FUNCTION "SFOGLIATORE" : VOID
TITLE =COMANDO SFOGLIATORE
AUTHOR : LD
FAMILY : DESTACK
NAME : SFOGL
VERSION : 0.1

BEGIN
NETWORK
TITLE =Sicurezze per sfogliatore
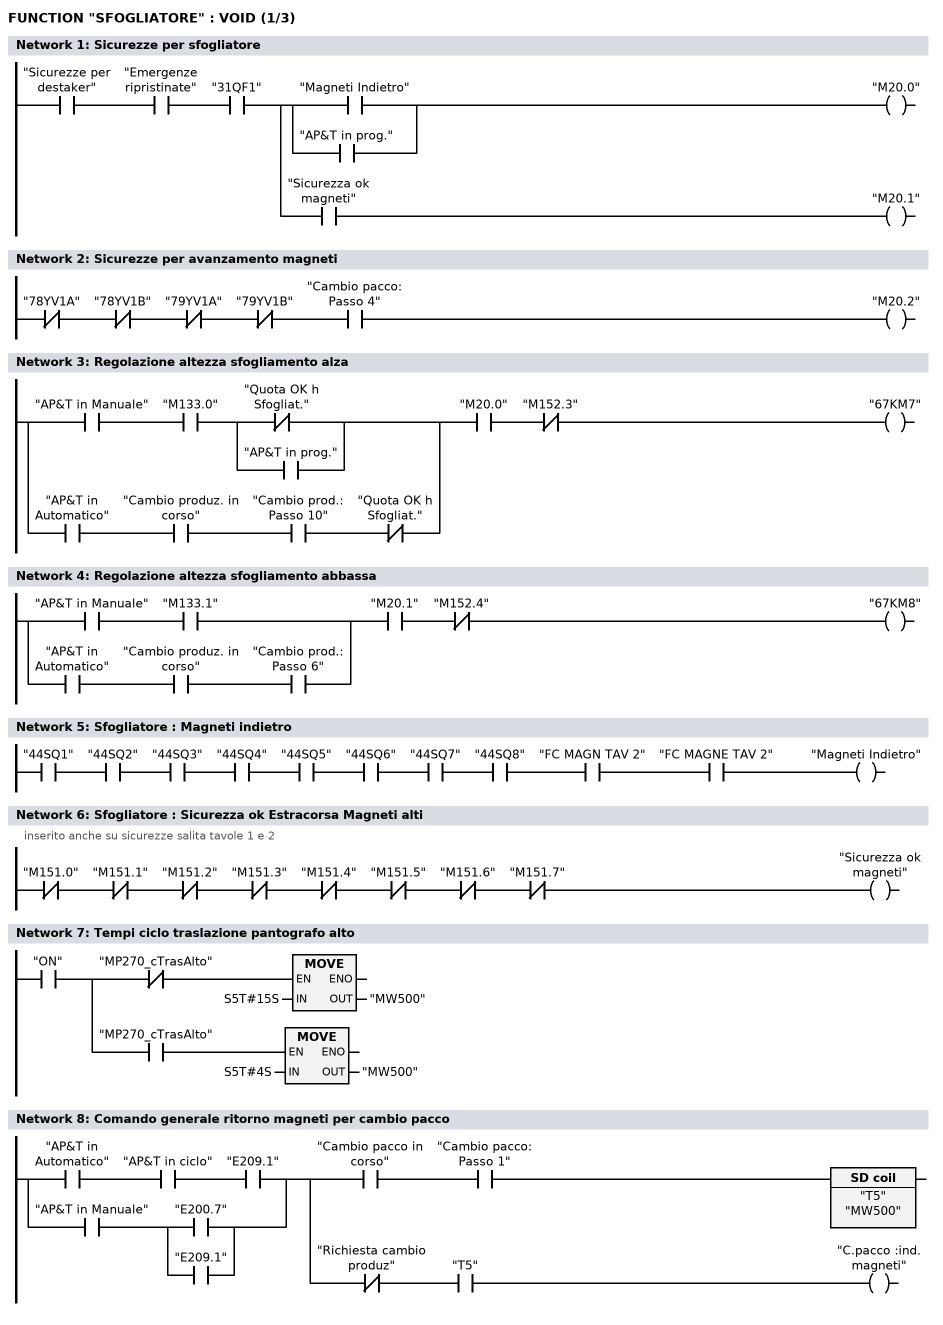
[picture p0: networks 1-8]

      U     "Sicurezze per destaker";
      U     "Emergenze ripristinate";
      U     "31QF1";
      =     L      0.0;
      U     L      0.0;
      U(    ;
      O     "Magneti Indietro";
      O     "AP&T in prog.";
      )     ;
      =     "M20.0";
      U     L      0.0;
      U     "Sicurezza ok magneti";
      =     "M20.1";
NETWORK
TITLE =Sicurezze per avanzamento magneti

      UN    "78YV1A";
      UN    "78YV1B";
      UN    "79YV1A";
      UN    "79YV1B";
      U     "Cambio pacco: Passo 4";
      =     "M20.2";
NETWORK
TITLE =Regolazione altezza sfogliamento alza

      U(    ;
      U     "AP&T in Manuale";
      U     "M133.0";
      U(    ;
      ON    "Quota OK h Sfogliat.";
      O     "AP&T in prog.";
      )     ;
      O     ;
      U     "AP&T in Automatico";
      U     "Cambio produz. in corso";
      U     "Cambio prod.: Passo 10";
      UN    "Quota OK h Sfogliat.";
      )     ;
      U     "M20.0";
      UN    "M152.3";
      =     "67KM7";
NETWORK
TITLE =Regolazione altezza sfogliamento abbassa

      U(    ;
      U     "AP&T in Manuale";
      U     "M133.1";
      O     ;
      U     "AP&T in Automatico";
      U     "Cambio produz. in corso";
      U     "Cambio prod.: Passo 6";
      )     ;
      U     "M20.1";
      UN    "M152.4";
      =     "67KM8";
NETWORK
TITLE =Sfogliatore : Magneti indietro

      U     "44SQ1";
      U     "44SQ2";
      U     "44SQ3";
      U     "44SQ4";
      U     "44SQ5";
      U     "44SQ6";
      U     "44SQ7";
      U     "44SQ8";
      U     "FC MAGN TAV 2";
      U     "FC MAGNE TAV 2";
      =     "Magneti Indietro";
NETWORK
TITLE =Sfogliatore : Sicurezza ok Estracorsa Magneti alti
//inserito anche su sicurezze salita tavole 1 e 2
      UN    "M151.0";
      UN    "M151.1";
      UN    "M151.2";
      UN    "M151.3";
      UN    "M151.4";
      UN    "M151.5";
      UN    "M151.6";
      UN    "M151.7";
      =     "Sicurezza ok magneti";
NETWORK
TITLE =Tempi ciclo traslazione pantografo alto

      U     "ON";
      =     L      0.0;
      U     L      0.0;
      UN    "MP270_cTrasAlto";
      SPBNB _001;
      L     S5T#15S;
      T     "MW500";
_001: NOP   0;
      U     L      0.0;
      U     "MP270_cTrasAlto";
      SPBNB _002;
      L     S5T#4S;
      T     "MW500";
_002: NOP   0;
NETWORK
TITLE =Comando generale ritorno magneti per cambio pacco

      U     "AP&T in Automatico";
      U     "AP&T in ciclo";
      U     "E209.1";
      O     ;
      U     "AP&T in Manuale";
      U(    ;
      O     "E200.7";
      O     "E209.1";
      )     ;
      =     L      0.0;
      U     L      0.0;
      U     "Cambio pacco in corso";
      U     "Cambio pacco: Passo 1";
      L     "MW500";
      SE    "T5";
      U     L      0.0;
      UN    "Richiesta cambio produz";
      U     "T5";
      =     "C.pacco :ind. magneti";
NETWORK
TITLE =Sfogliatore : Comando Impulso vuoto per ripristino prelievo
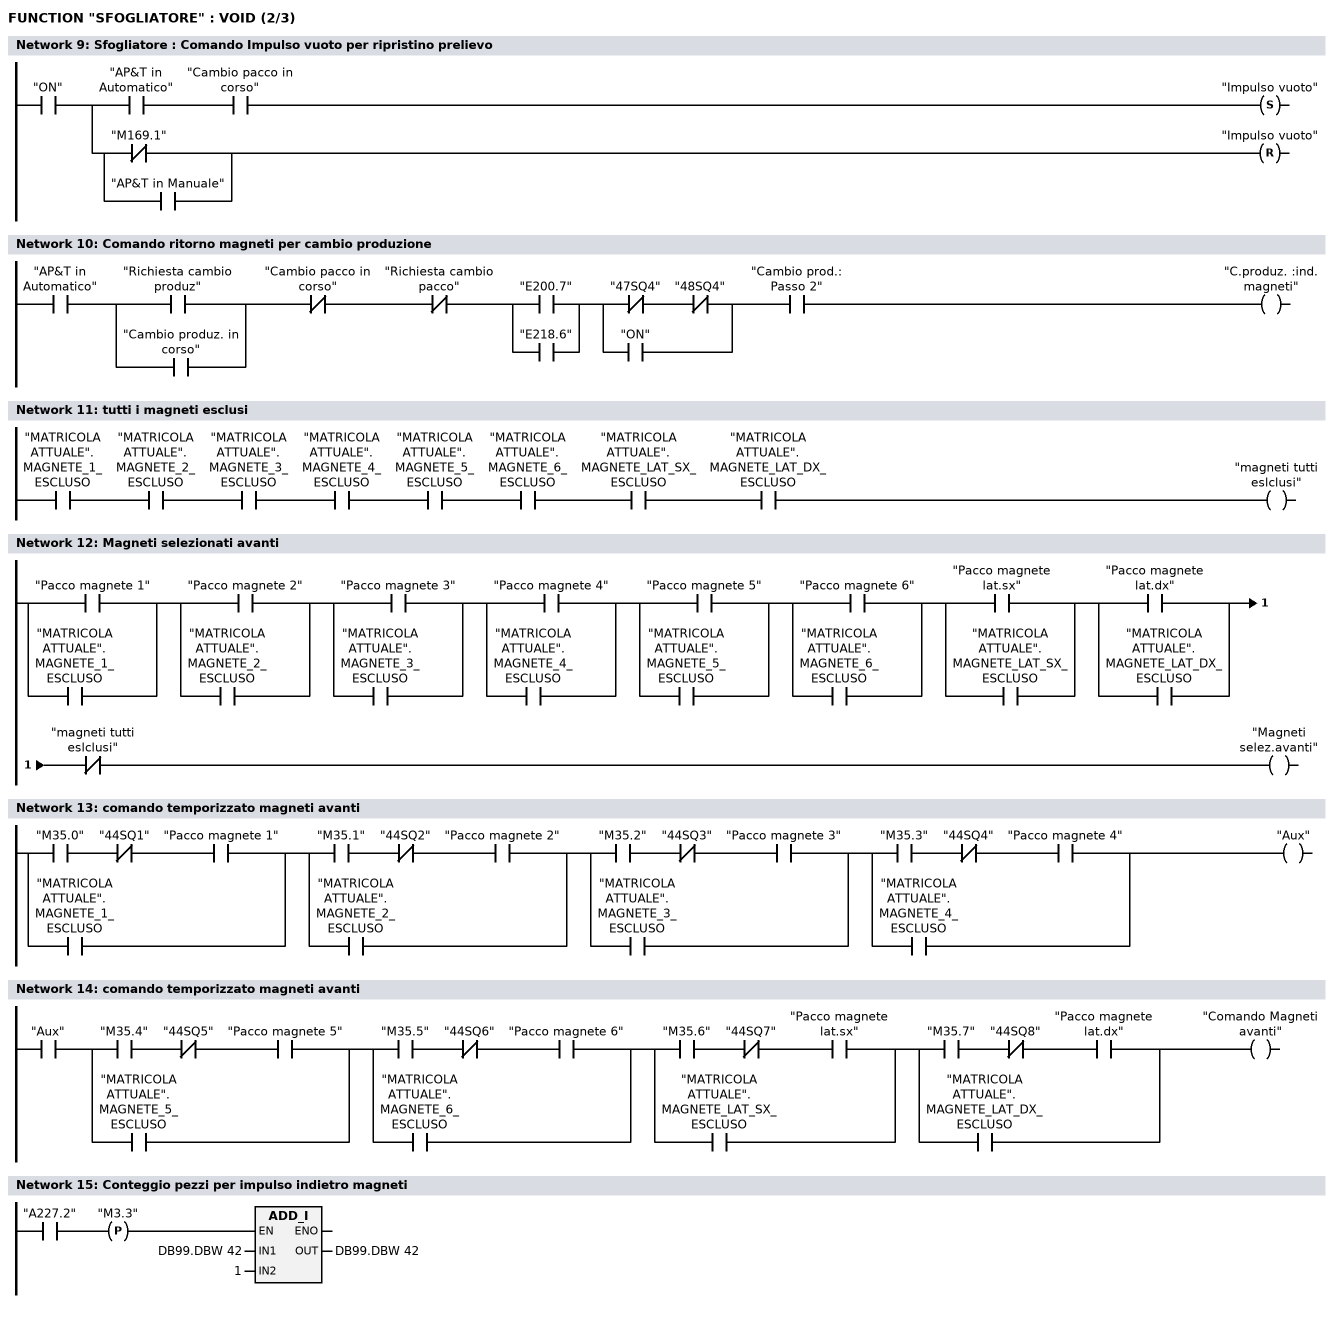
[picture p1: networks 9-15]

      U     "ON";
      =     L      0.0;
      U     L      0.0;
      U     "AP&T in Automatico";
      U     "Cambio pacco in corso";
      S     "Impulso vuoto";
      U     L      0.0;
      U(    ;
      ON    "M169.1";
      O     "AP&T in Manuale";
      )     ;
      R     "Impulso vuoto";
NETWORK
TITLE =Comando ritorno magneti per cambio produzione

      U     "AP&T in Automatico";
      U(    ;
      O     "Richiesta cambio produz";
      O     "Cambio produz. in corso";
      )     ;
      UN    "Cambio pacco in corso";
      UN    "Richiesta cambio pacco";
      U(    ;
      O     "E200.7";
      O     "E218.6";
      )     ;
      U(    ;
      UN    "47SQ4";
      UN    "48SQ4";
      O     "ON";
      )     ;
      U     "Cambio prod.: Passo 2";
      =     "C.produz. :ind. magneti";
NETWORK
TITLE =tutti i magneti esclusi



      U     "MATRICOLA ATTUALE".MAGNETE_1_ESCLUSO;
      U     "MATRICOLA ATTUALE".MAGNETE_2_ESCLUSO;
      U     "MATRICOLA ATTUALE".MAGNETE_3_ESCLUSO;
      U     "MATRICOLA ATTUALE".MAGNETE_4_ESCLUSO;
      U     "MATRICOLA ATTUALE".MAGNETE_5_ESCLUSO;
      U     "MATRICOLA ATTUALE".MAGNETE_6_ESCLUSO;
      U     "MATRICOLA ATTUALE".MAGNETE_LAT_SX_ESCLUSO;
      U     "MATRICOLA ATTUALE".MAGNETE_LAT_DX_ESCLUSO;
      =     "magneti tutti eslclusi";
NETWORK
TITLE =Magneti selezionati avanti

      U(    ;
      O     "Pacco magnete 1";
      O     "MATRICOLA ATTUALE".MAGNETE_1_ESCLUSO;
      )     ;
      U(    ;
      O     "Pacco magnete 2";
      O     "MATRICOLA ATTUALE".MAGNETE_2_ESCLUSO;
      )     ;
      U(    ;
      O     "Pacco magnete 3";
      O     "MATRICOLA ATTUALE".MAGNETE_3_ESCLUSO;
      )     ;
      U(    ;
      O     "Pacco magnete 4";
      O     "MATRICOLA ATTUALE".MAGNETE_4_ESCLUSO;
      )     ;
      U(    ;
      O     "Pacco magnete 5";
      O     "MATRICOLA ATTUALE".MAGNETE_5_ESCLUSO;
      )     ;
      U(    ;
      O     "Pacco magnete 6";
      O     "MATRICOLA ATTUALE".MAGNETE_6_ESCLUSO;
      )     ;
      U(    ;
      O     "Pacco magnete lat.sx";
      O     "MATRICOLA ATTUALE".MAGNETE_LAT_SX_ESCLUSO;
      )     ;
      U(    ;
      O     "Pacco magnete lat.dx";
      O     "MATRICOLA ATTUALE".MAGNETE_LAT_DX_ESCLUSO;
      )     ;
      UN    "magneti tutti eslclusi";
      =     "Magneti selez.avanti";
NETWORK
TITLE =comando temporizzato magneti avanti

      U(    ;
      U     "M35.0";
      UN    "44SQ1";
      U     "Pacco magnete 1";
      O     "MATRICOLA ATTUALE".MAGNETE_1_ESCLUSO;
      )     ;
      U(    ;
      U     "M35.1";
      UN    "44SQ2";
      U     "Pacco magnete 2";
      O     "MATRICOLA ATTUALE".MAGNETE_2_ESCLUSO;
      )     ;
      U(    ;
      U     "M35.2";
      UN    "44SQ3";
      U     "Pacco magnete 3";
      O     "MATRICOLA ATTUALE".MAGNETE_3_ESCLUSO;
      )     ;
      U(    ;
      U     "M35.3";
      UN    "44SQ4";
      U     "Pacco magnete 4";
      O     "MATRICOLA ATTUALE".MAGNETE_4_ESCLUSO;
      )     ;
      =     "Aux";
NETWORK
TITLE =comando temporizzato magneti avanti

      U     "Aux";
      U(    ;
      U     "M35.4";
      UN    "44SQ5";
      U     "Pacco magnete 5";
      O     "MATRICOLA ATTUALE".MAGNETE_5_ESCLUSO;
      )     ;
      U(    ;
      U     "M35.5";
      UN    "44SQ6";
      U     "Pacco magnete 6";
      O     "MATRICOLA ATTUALE".MAGNETE_6_ESCLUSO;
      )     ;
      U(    ;
      U     "M35.6";
      UN    "44SQ7";
      U     "Pacco magnete lat.sx";
      O     "MATRICOLA ATTUALE".MAGNETE_LAT_SX_ESCLUSO;
      )     ;
      U(    ;
      U     "M35.7";
      UN    "44SQ8";
      U     "Pacco magnete lat.dx";
      O     "MATRICOLA ATTUALE".MAGNETE_LAT_DX_ESCLUSO;
      )     ;
      =     "Comando Magneti avanti";
NETWORK
TITLE =Conteggio pezzi per impulso indietro magneti

      U     "A227.2";
      FP    "M3.3";
      SPBNB _003;
      L     DB99.DBW   42;
      L     1;
      +I    ;
      T     DB99.DBW   42;
_003: NOP   0;
NETWORK
TITLE =Aux impulso per magneti indietro
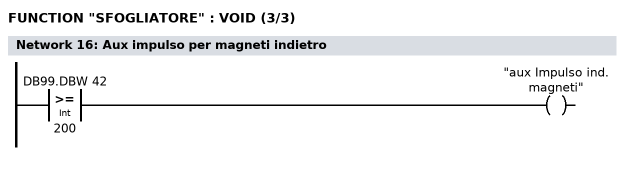
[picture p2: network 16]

      L     DB99.DBW   42;
      L     200;
      >=I   ;
      =     "aux Impulso ind. magneti";
NETWORK
TITLE =Memoria magneti avanti

      U(    ;
      O     "Comando Magneti avanti";
      O(    ;
      U     "Cambio pacco in corso";
      U     "Cambio pacco: Passo 4";
      UN    "Magneti Indietro";
      L     S5T#10S;
      SE    "T12";
      NOP   0;
      NOP   0;
      NOP   0;
      U     "T12";
      )     ;
      O     ;
      U(    ;
      O     "AP&T in Manuale";
      O     "Singolo";
      )     ;
      UN    "Cambio pacco in corso";
      UN    "Magneti Indietro";
      )     ;
      S     "M39.5";
      U     "Magneti Indietro";
      R     "M39.5";
      U     "M39.5";
      L     S5T#100MS;
      SE    "T6";
NETWORK
TITLE =
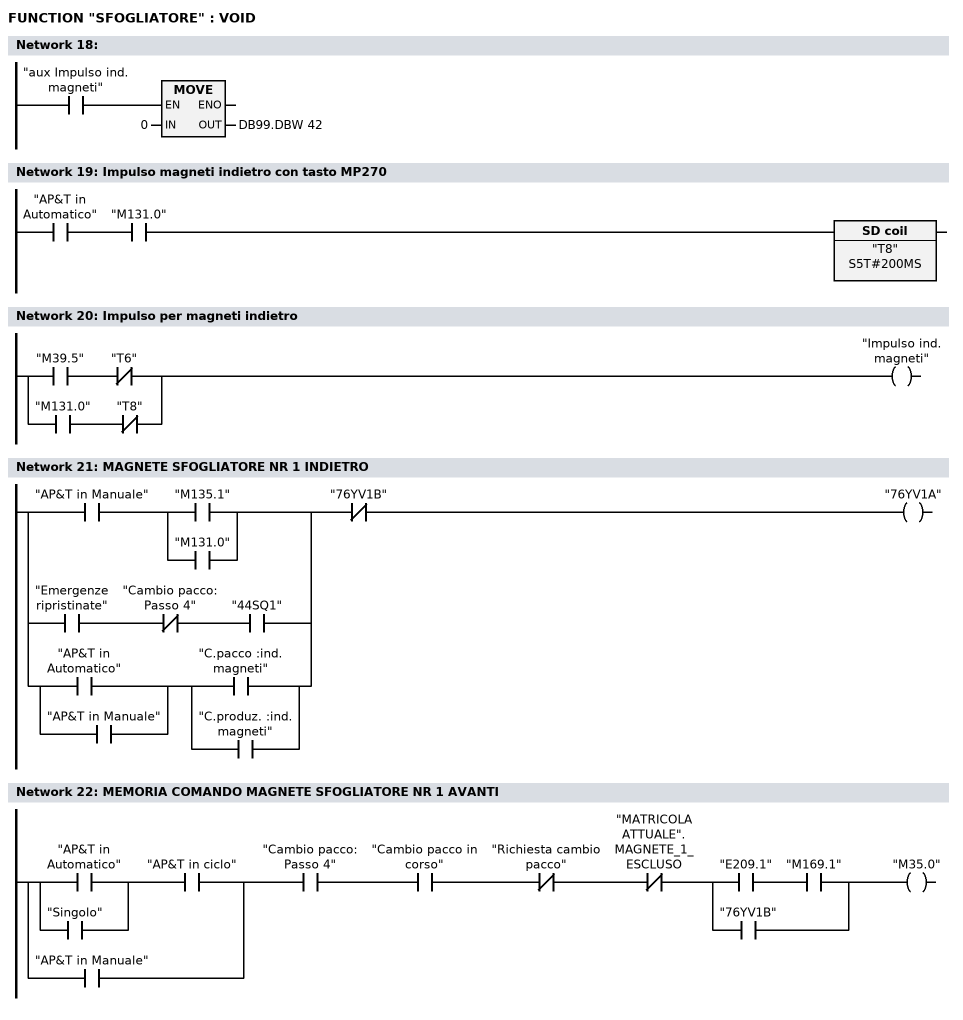
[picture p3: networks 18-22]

      U     "aux Impulso ind. magneti";
      SPBNB _004;
      L     0;
      T     DB99.DBW   42;
_004: NOP   0;
NETWORK
TITLE =Impulso magneti indietro con tasto MP270

      U     "AP&T in Automatico";
      U     "M131.0";
      L     S5T#200MS;
      SE    "T8";
NETWORK
TITLE =Impulso per magneti indietro

      U     "M39.5";
      UN    "T6";
      O     ;
      U     "M131.0";
      UN    "T8";
      =     "Impulso ind. magneti";
NETWORK
TITLE =MAGNETE SFOGLIATORE NR 1 INDIETRO

      U(    ;
      U     "AP&T in Manuale";
      U(    ;
      O     "M135.1";
      O     "M131.0";
      )     ;
      O     ;
      U     "Emergenze ripristinate";
      UN    "Cambio pacco: Passo 4";
      U     "44SQ1";
      O     ;
      U(    ;
      O     "AP&T in Automatico";
      O     "AP&T in Manuale";
      )     ;
      U(    ;
      O     "C.pacco :ind. magneti";
      O     "C.produz. :ind. magneti";
      )     ;
      )     ;
      UN    "76YV1B";
      =     "76YV1A";
NETWORK
TITLE =MEMORIA COMANDO MAGNETE SFOGLIATORE NR 1 AVANTI

      U(    ;
      U(    ;
      O     "AP&T in Automatico";
      O     "Singolo";
      )     ;
      U     "AP&T in ciclo";
      O     "AP&T in Manuale";
      )     ;
      U     "Cambio pacco: Passo 4";
      U     "Cambio pacco in corso";
      UN    "Richiesta cambio pacco";
      UN    "MATRICOLA ATTUALE".MAGNETE_1_ESCLUSO;
      U(    ;
      U     "E209.1";
      U     "M169.1";
      O     "76YV1B";
      )     ;
      =     "M35.0";
NETWORK
TITLE =COMANDO MAGNETE SFOGLIATORE NR 1 AVANTI

      O(    ;
      U(    ;
      U(    ;
      O     "AP&T in Automatico";
      O     "Singolo";
      )     ;
      U     "AP&T in ciclo";
      O     "AP&T in Manuale";
      )     ;
      U     "M35.0";
      U     "M20.2";
      UN    "Pacco magnete 1";
      L     S5T#500MS;
      SA    "M1_RitAvanti";
      NOP   0;
      NOP   0;
      NOP   0;
      U     "M1_RitAvanti";
      )     ;
      O     ;
      U(    ;
      O     "AP&T in Manuale";
      O     "AP&T in prog.";
      )     ;
      U(    ;
      O     "M135.0";
      O     ;
      U     "M137.4";
      UN    "MATRICOLA ATTUALE".MAGNETE_1_ESCLUSO;
      )     ;
      =     "76YV1B";
NETWORK
TITLE =MAGNETE SFOGLIATORE NR 2 INDIETRO
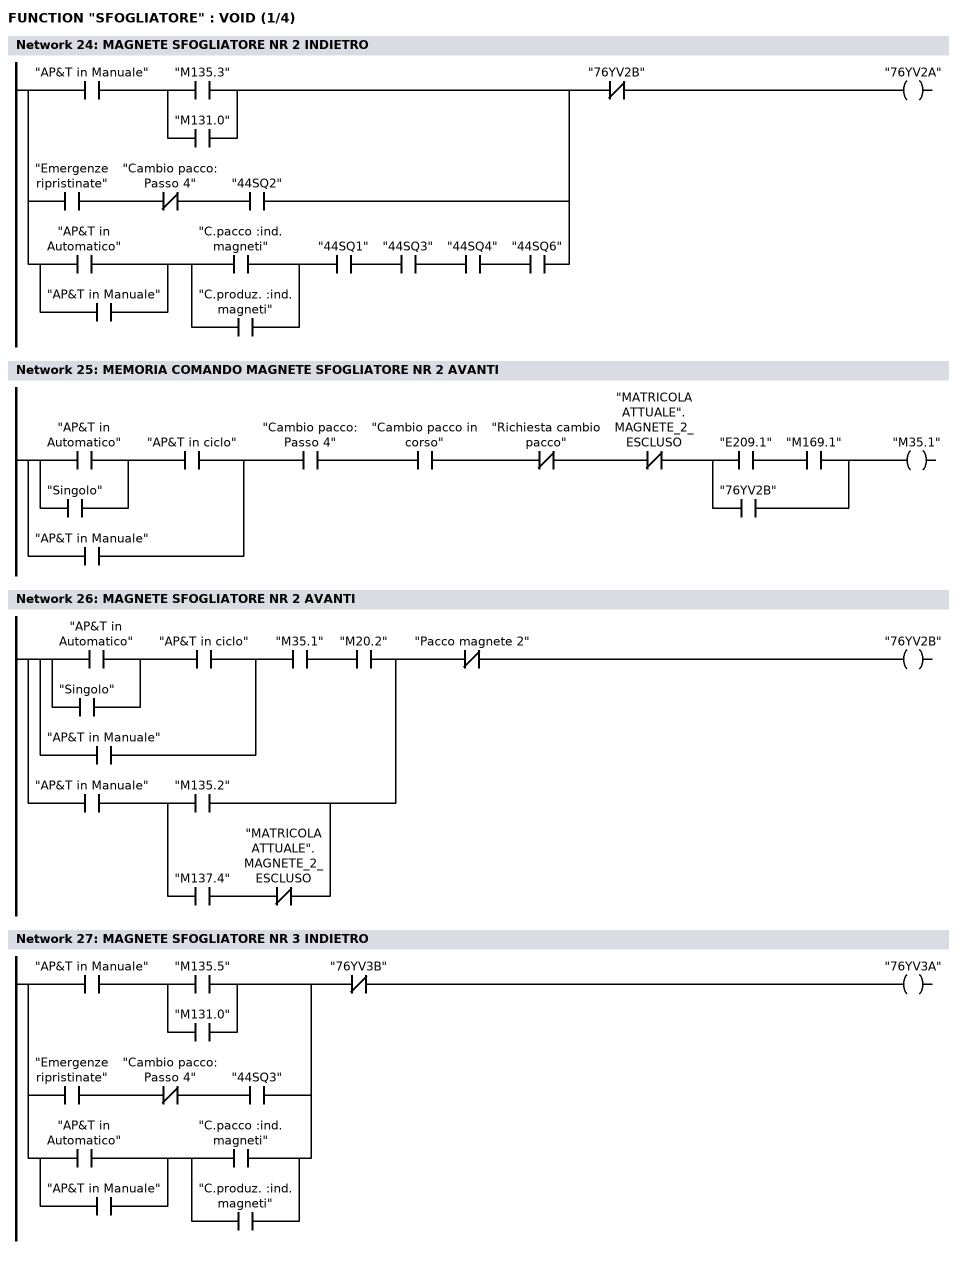
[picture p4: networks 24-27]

      U(    ;
      U     "AP&T in Manuale";
      U(    ;
      O     "M135.3";
      O     "M131.0";
      )     ;
      O     ;
      U     "Emergenze ripristinate";
      UN    "Cambio pacco: Passo 4";
      U     "44SQ2";
      O     ;
      U(    ;
      O     "AP&T in Automatico";
      O     "AP&T in Manuale";
      )     ;
      U(    ;
      O     "C.pacco :ind. magneti";
      O     "C.produz. :ind. magneti";
      )     ;
      U     "44SQ1";
      U     "44SQ3";
      U     "44SQ4";
      U     "44SQ6";
      )     ;
      UN    "76YV2B";
      =     "76YV2A";
NETWORK
TITLE =MEMORIA COMANDO MAGNETE SFOGLIATORE NR 2 AVANTI

      U(    ;
      U(    ;
      O     "AP&T in Automatico";
      O     "Singolo";
      )     ;
      U     "AP&T in ciclo";
      O     "AP&T in Manuale";
      )     ;
      U     "Cambio pacco: Passo 4";
      U     "Cambio pacco in corso";
      UN    "Richiesta cambio pacco";
      UN    "MATRICOLA ATTUALE".MAGNETE_2_ESCLUSO;
      U(    ;
      U     "E209.1";
      U     "M169.1";
      O     "76YV2B";
      )     ;
      =     "M35.1";
NETWORK
TITLE =MAGNETE SFOGLIATORE NR 2 AVANTI

      U(    ;
      U(    ;
      U(    ;
      O     "AP&T in Automatico";
      O     "Singolo";
      )     ;
      U     "AP&T in ciclo";
      O     "AP&T in Manuale";
      )     ;
      U     "M35.1";
      U     "M20.2";
      O     ;
      U     "AP&T in Manuale";
      U(    ;
      O     "M135.2";
      O     ;
      U     "M137.4";
      UN    "MATRICOLA ATTUALE".MAGNETE_2_ESCLUSO;
      )     ;
      )     ;
      UN    "Pacco magnete 2";
      =     "76YV2B";
NETWORK
TITLE =MAGNETE SFOGLIATORE NR 3 INDIETRO

      U(    ;
      U     "AP&T in Manuale";
      U(    ;
      O     "M135.5";
      O     "M131.0";
      )     ;
      O     ;
      U     "Emergenze ripristinate";
      UN    "Cambio pacco: Passo 4";
      U     "44SQ3";
      O     ;
      U(    ;
      O     "AP&T in Automatico";
      O     "AP&T in Manuale";
      )     ;
      U(    ;
      O     "C.pacco :ind. magneti";
      O     "C.produz. :ind. magneti";
      )     ;
      )     ;
      UN    "76YV3B";
      =     "76YV3A";
NETWORK
TITLE =MEMORIA COMANDO MAGNETE SFOGLIATORE NR 3 AVANTI
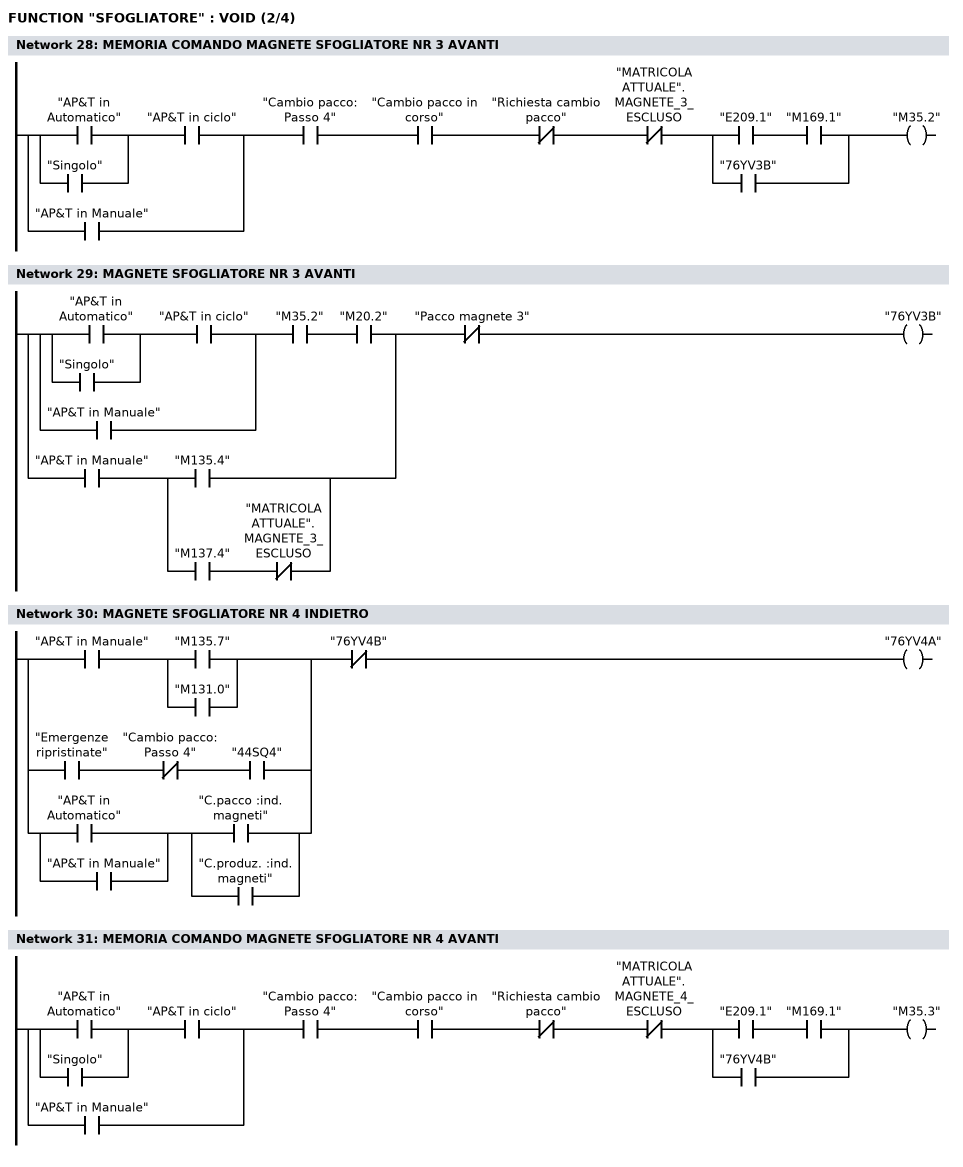
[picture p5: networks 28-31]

      U(    ;
      U(    ;
      O     "AP&T in Automatico";
      O     "Singolo";
      )     ;
      U     "AP&T in ciclo";
      O     "AP&T in Manuale";
      )     ;
      U     "Cambio pacco: Passo 4";
      U     "Cambio pacco in corso";
      UN    "Richiesta cambio pacco";
      UN    "MATRICOLA ATTUALE".MAGNETE_3_ESCLUSO;
      U(    ;
      U     "E209.1";
      U     "M169.1";
      O     "76YV3B";
      )     ;
      =     "M35.2";
NETWORK
TITLE =MAGNETE SFOGLIATORE NR 3 AVANTI

      U(    ;
      U(    ;
      U(    ;
      O     "AP&T in Automatico";
      O     "Singolo";
      )     ;
      U     "AP&T in ciclo";
      O     "AP&T in Manuale";
      )     ;
      U     "M35.2";
      U     "M20.2";
      O     ;
      U     "AP&T in Manuale";
      U(    ;
      O     "M135.4";
      O     ;
      U     "M137.4";
      UN    "MATRICOLA ATTUALE".MAGNETE_3_ESCLUSO;
      )     ;
      )     ;
      UN    "Pacco magnete 3";
      =     "76YV3B";
NETWORK
TITLE =MAGNETE SFOGLIATORE NR 4 INDIETRO

      U(    ;
      U     "AP&T in Manuale";
      U(    ;
      O     "M135.7";
      O     "M131.0";
      )     ;
      O     ;
      U     "Emergenze ripristinate";
      UN    "Cambio pacco: Passo 4";
      U     "44SQ4";
      O     ;
      U(    ;
      O     "AP&T in Automatico";
      O     "AP&T in Manuale";
      )     ;
      U(    ;
      O     "C.pacco :ind. magneti";
      O     "C.produz. :ind. magneti";
      )     ;
      )     ;
      UN    "76YV4B";
      =     "76YV4A";
NETWORK
TITLE =MEMORIA COMANDO MAGNETE SFOGLIATORE NR 4 AVANTI

      U(    ;
      U(    ;
      O     "AP&T in Automatico";
      O     "Singolo";
      )     ;
      U     "AP&T in ciclo";
      O     "AP&T in Manuale";
      )     ;
      U     "Cambio pacco: Passo 4";
      U     "Cambio pacco in corso";
      UN    "Richiesta cambio pacco";
      UN    "MATRICOLA ATTUALE".MAGNETE_4_ESCLUSO;
      U(    ;
      U     "E209.1";
      U     "M169.1";
      O     "76YV4B";
      )     ;
      =     "M35.3";
NETWORK
TITLE =MAGNETE SFOGLIATORE NR 4 AVANTI
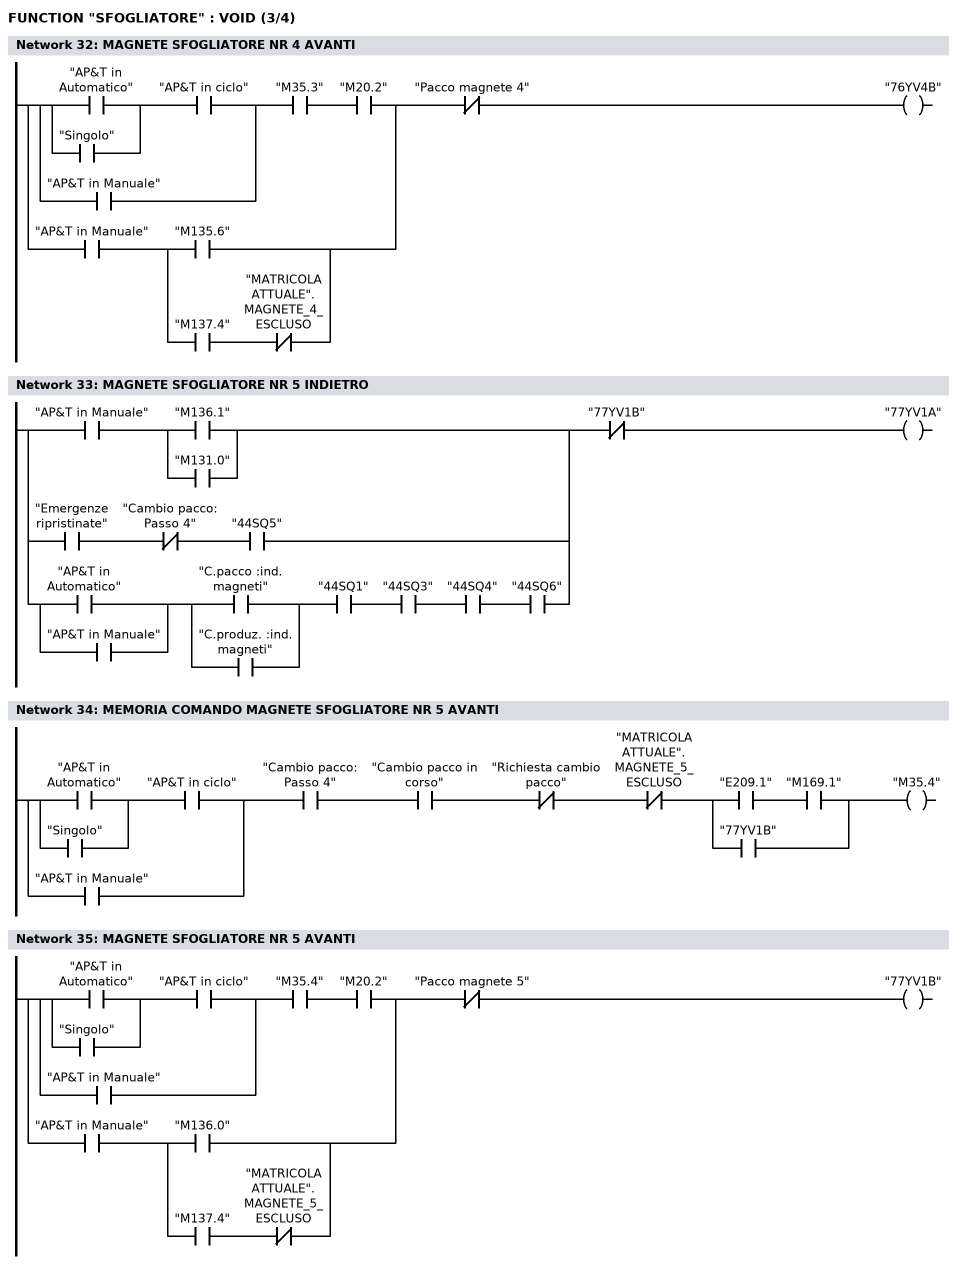
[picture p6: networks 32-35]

      U(    ;
      U(    ;
      U(    ;
      O     "AP&T in Automatico";
      O     "Singolo";
      )     ;
      U     "AP&T in ciclo";
      O     "AP&T in Manuale";
      )     ;
      U     "M35.3";
      U     "M20.2";
      O     ;
      U     "AP&T in Manuale";
      U(    ;
      O     "M135.6";
      O     ;
      U     "M137.4";
      UN    "MATRICOLA ATTUALE".MAGNETE_4_ESCLUSO;
      )     ;
      )     ;
      UN    "Pacco magnete 4";
      =     "76YV4B";
NETWORK
TITLE =MAGNETE SFOGLIATORE NR 5 INDIETRO

      U(    ;
      U     "AP&T in Manuale";
      U(    ;
      O     "M136.1";
      O     "M131.0";
      )     ;
      O     ;
      U     "Emergenze ripristinate";
      UN    "Cambio pacco: Passo 4";
      U     "44SQ5";
      O     ;
      U(    ;
      O     "AP&T in Automatico";
      O     "AP&T in Manuale";
      )     ;
      U(    ;
      O     "C.pacco :ind. magneti";
      O     "C.produz. :ind. magneti";
      )     ;
      U     "44SQ1";
      U     "44SQ3";
      U     "44SQ4";
      U     "44SQ6";
      )     ;
      UN    "77YV1B";
      =     "77YV1A";
NETWORK
TITLE =MEMORIA COMANDO MAGNETE SFOGLIATORE NR 5 AVANTI

      U(    ;
      U(    ;
      O     "AP&T in Automatico";
      O     "Singolo";
      )     ;
      U     "AP&T in ciclo";
      O     "AP&T in Manuale";
      )     ;
      U     "Cambio pacco: Passo 4";
      U     "Cambio pacco in corso";
      UN    "Richiesta cambio pacco";
      UN    "MATRICOLA ATTUALE".MAGNETE_5_ESCLUSO;
      U(    ;
      U     "E209.1";
      U     "M169.1";
      O     "77YV1B";
      )     ;
      =     "M35.4";
NETWORK
TITLE =MAGNETE SFOGLIATORE NR 5 AVANTI

      U(    ;
      U(    ;
      U(    ;
      O     "AP&T in Automatico";
      O     "Singolo";
      )     ;
      U     "AP&T in ciclo";
      O     "AP&T in Manuale";
      )     ;
      U     "M35.4";
      U     "M20.2";
      O     ;
      U     "AP&T in Manuale";
      U(    ;
      O     "M136.0";
      O     ;
      U     "M137.4";
      UN    "MATRICOLA ATTUALE".MAGNETE_5_ESCLUSO;
      )     ;
      )     ;
      UN    "Pacco magnete 5";
      =     "77YV1B";
NETWORK
TITLE =MAGNETE SFOGLIATORE NR 6 INDIETRO
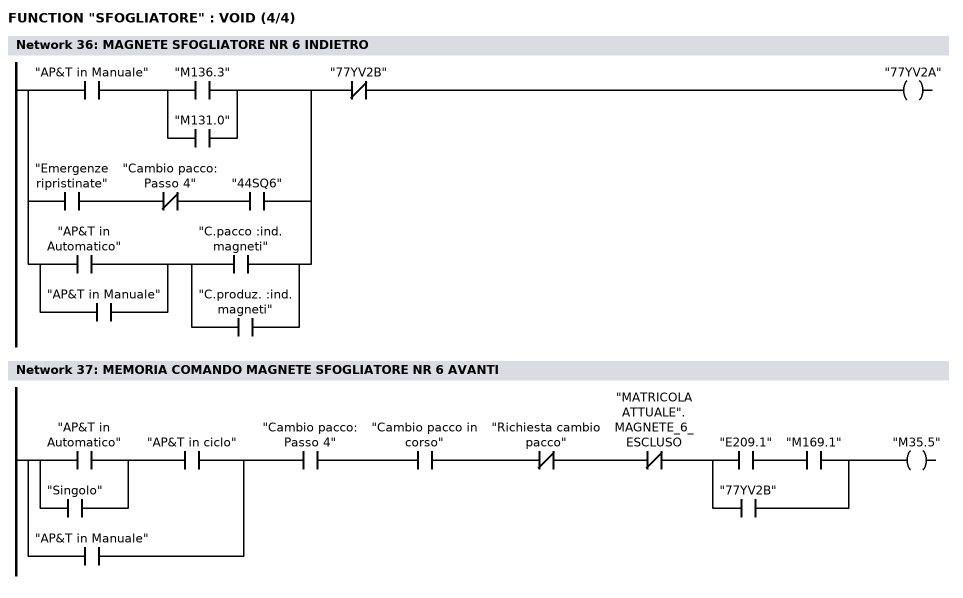
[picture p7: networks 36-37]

      U(    ;
      U     "AP&T in Manuale";
      U(    ;
      O     "M136.3";
      O     "M131.0";
      )     ;
      O     ;
      U     "Emergenze ripristinate";
      UN    "Cambio pacco: Passo 4";
      U     "44SQ6";
      O     ;
      U(    ;
      O     "AP&T in Automatico";
      O     "AP&T in Manuale";
      )     ;
      U(    ;
      O     "C.pacco :ind. magneti";
      O     "C.produz. :ind. magneti";
      )     ;
      )     ;
      UN    "77YV2B";
      =     "77YV2A";
NETWORK
TITLE =MEMORIA COMANDO MAGNETE SFOGLIATORE NR 6 AVANTI

      U(    ;
      U(    ;
      O     "AP&T in Automatico";
      O     "Singolo";
      )     ;
      U     "AP&T in ciclo";
      O     "AP&T in Manuale";
      )     ;
      U     "Cambio pacco: Passo 4";
      U     "Cambio pacco in corso";
      UN    "Richiesta cambio pacco";
      UN    "MATRICOLA ATTUALE".MAGNETE_6_ESCLUSO;
      U(    ;
      U     "E209.1";
      U     "M169.1";
      O     "77YV2B";
      )     ;
      =     "M35.5";
NETWORK
TITLE =MAGNETE SFOGLIATORE NR 6 AVANTI

      O(    ;
      U(    ;
      U(    ;
      O     "AP&T in Automatico";
      O     "Singolo";
      )     ;
      U     "AP&T in ciclo";
      O     "AP&T in Manuale";
      )     ;
      U     "M35.5";
      U     "M20.2";
      UN    "Pacco magnete 6";
      L     S5T#3S;
      SA    "M6_RitAvanti";
      NOP   0;
      NOP   0;
      NOP   0;
      U     "M6_RitAvanti";
      )     ;
      O     ;
      U(    ;
      O     "AP&T in Manuale";
      O     "AP&T in prog.";
      )     ;
      U(    ;
      O     "M136.2";
      O     ;
      U     "M137.4";
      UN    "MATRICOLA ATTUALE".MAGNETE_6_ESCLUSO;
      )     ;
      =     "77YV2B";
NETWORK
TITLE =MAGNETE SFOGLIATORE LATERALE SX INDIETRO
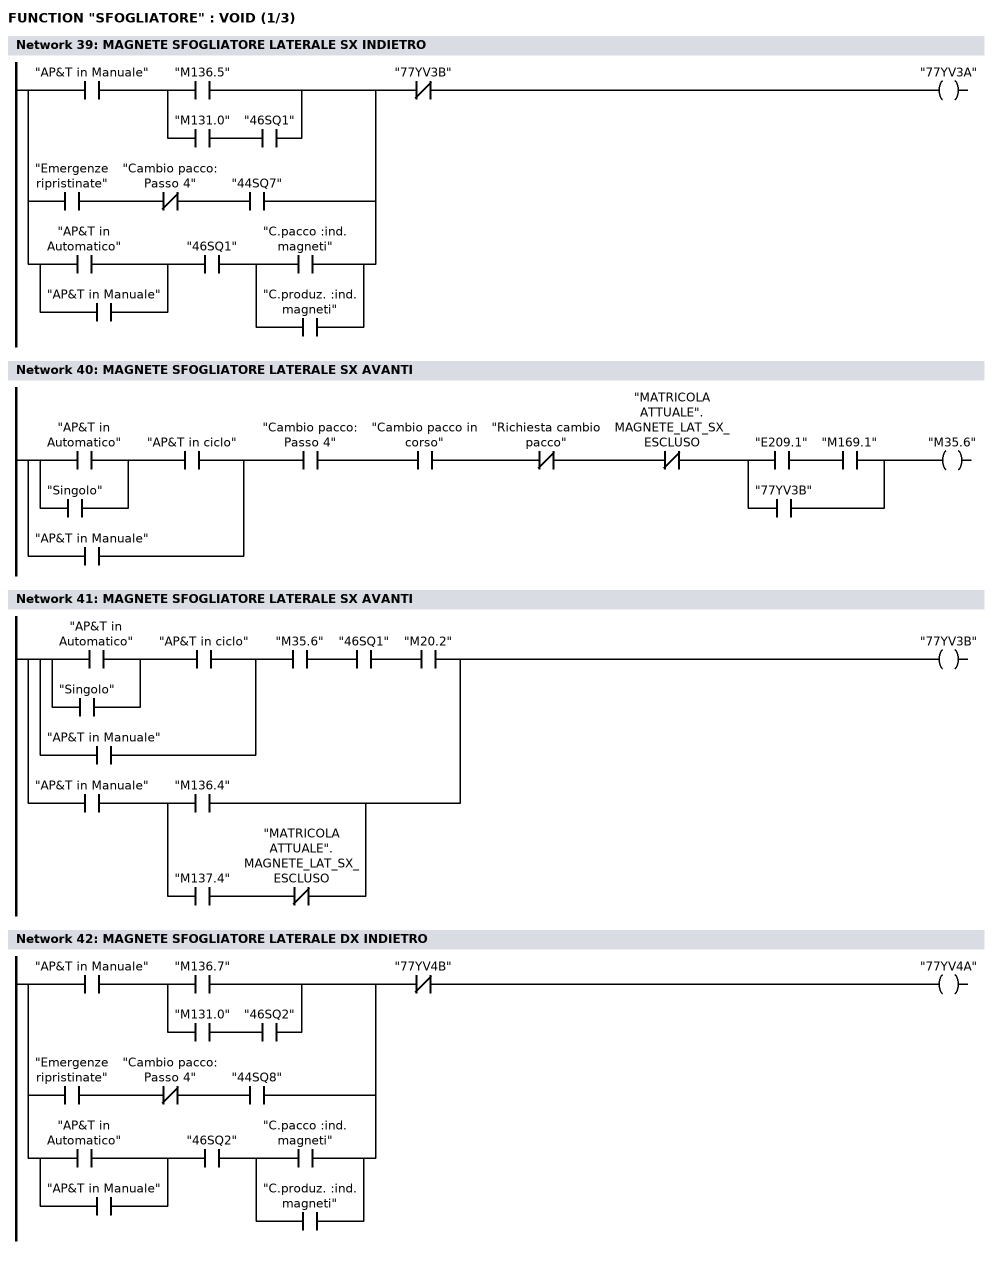
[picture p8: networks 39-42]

      U(    ;
      U     "AP&T in Manuale";
      U(    ;
      O     "M136.5";
      O     ;
      U     "M131.0";
      U     "46SQ1";
      )     ;
      O     ;
      U     "Emergenze ripristinate";
      UN    "Cambio pacco: Passo 4";
      U     "44SQ7";
      O     ;
      U(    ;
      O     "AP&T in Automatico";
      O     "AP&T in Manuale";
      )     ;
      U     "46SQ1";
      U(    ;
      O     "C.pacco :ind. magneti";
      O     "C.produz. :ind. magneti";
      )     ;
      )     ;
      UN    "77YV3B";
      =     "77YV3A";
NETWORK
TITLE =MAGNETE SFOGLIATORE LATERALE SX AVANTI

      U(    ;
      U(    ;
      O     "AP&T in Automatico";
      O     "Singolo";
      )     ;
      U     "AP&T in ciclo";
      O     "AP&T in Manuale";
      )     ;
      U     "Cambio pacco: Passo 4";
      U     "Cambio pacco in corso";
      UN    "Richiesta cambio pacco";
      UN    "MATRICOLA ATTUALE".MAGNETE_LAT_SX_ESCLUSO;
      U(    ;
      U     "E209.1";
      U     "M169.1";
      O     "77YV3B";
      )     ;
      =     "M35.6";
NETWORK
TITLE =MAGNETE SFOGLIATORE LATERALE SX AVANTI

      U(    ;
      U(    ;
      O     "AP&T in Automatico";
      O     "Singolo";
      )     ;
      U     "AP&T in ciclo";
      O     "AP&T in Manuale";
      )     ;
      U     "M35.6";
      U     "46SQ1";
      U     "M20.2";
      O     ;
      U     "AP&T in Manuale";
      U(    ;
      O     "M136.4";
      O     ;
      U     "M137.4";
      UN    "MATRICOLA ATTUALE".MAGNETE_LAT_SX_ESCLUSO;
      )     ;
      =     "77YV3B";
NETWORK
TITLE =MAGNETE SFOGLIATORE LATERALE DX INDIETRO

      U(    ;
      U     "AP&T in Manuale";
      U(    ;
      O     "M136.7";
      O     ;
      U     "M131.0";
      U     "46SQ2";
      )     ;
      O     ;
      U     "Emergenze ripristinate";
      UN    "Cambio pacco: Passo 4";
      U     "44SQ8";
      O     ;
      U(    ;
      O     "AP&T in Automatico";
      O     "AP&T in Manuale";
      )     ;
      U     "46SQ2";
      U(    ;
      O     "C.pacco :ind. magneti";
      O     "C.produz. :ind. magneti";
      )     ;
      )     ;
      UN    "77YV4B";
      =     "77YV4A";
NETWORK
TITLE =MAGNETE SFOGLIATORE LATERALE DX AVANTI
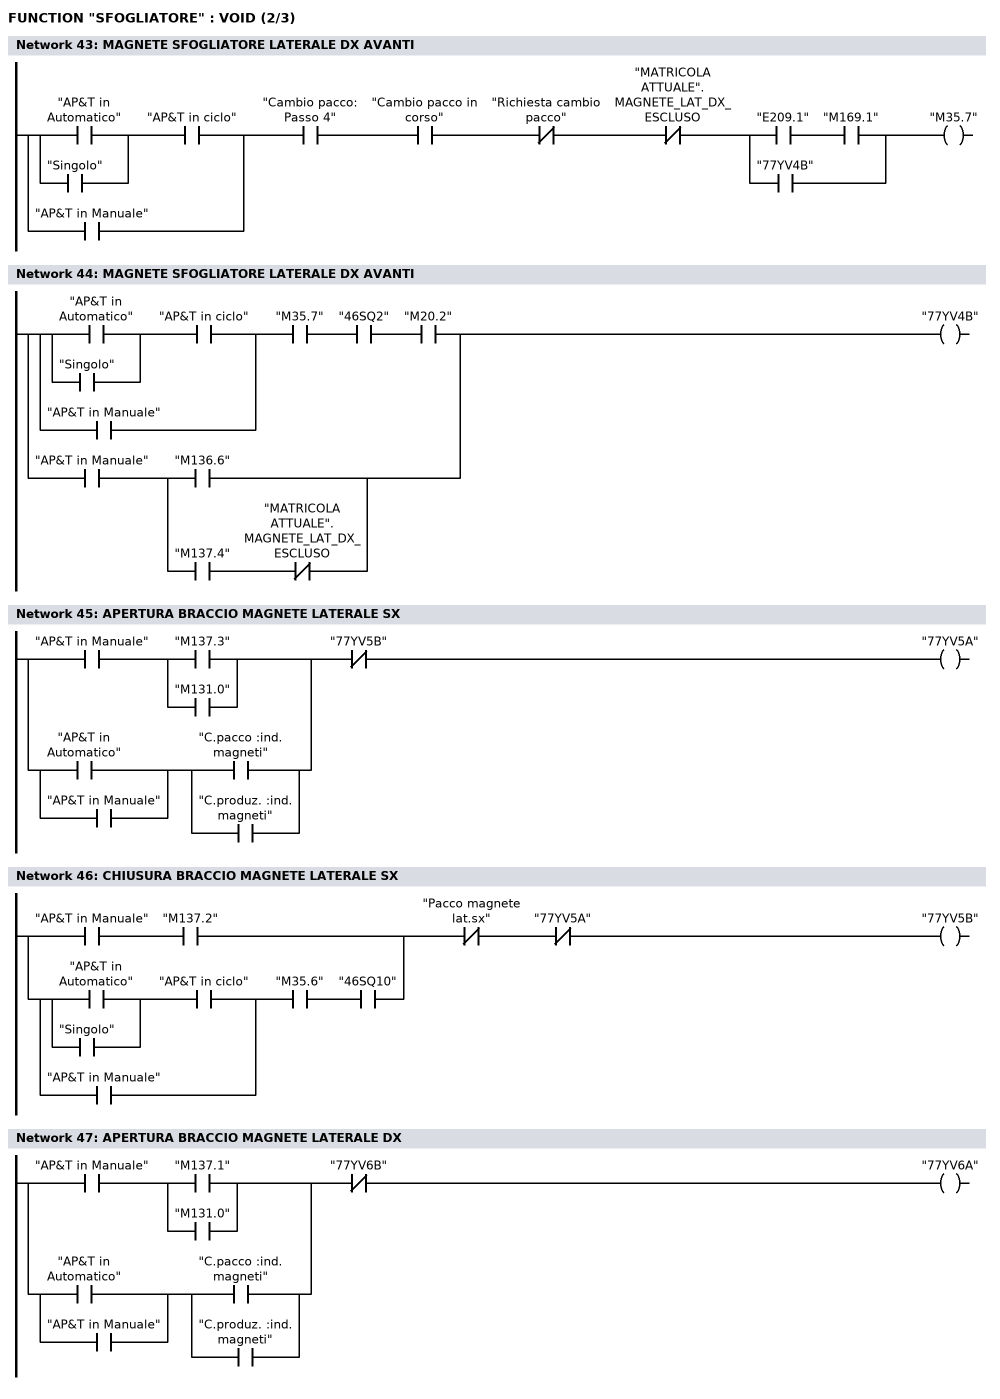
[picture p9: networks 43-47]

      U(    ;
      U(    ;
      O     "AP&T in Automatico";
      O     "Singolo";
      )     ;
      U     "AP&T in ciclo";
      O     "AP&T in Manuale";
      )     ;
      U     "Cambio pacco: Passo 4";
      U     "Cambio pacco in corso";
      UN    "Richiesta cambio pacco";
      UN    "MATRICOLA ATTUALE".MAGNETE_LAT_DX_ESCLUSO;
      U(    ;
      U     "E209.1";
      U     "M169.1";
      O     "77YV4B";
      )     ;
      =     "M35.7";
NETWORK
TITLE =MAGNETE SFOGLIATORE LATERALE DX AVANTI

      U(    ;
      U(    ;
      O     "AP&T in Automatico";
      O     "Singolo";
      )     ;
      U     "AP&T in ciclo";
      O     "AP&T in Manuale";
      )     ;
      U     "M35.7";
      U     "46SQ2";
      U     "M20.2";
      O     ;
      U     "AP&T in Manuale";
      U(    ;
      O     "M136.6";
      O     ;
      U     "M137.4";
      UN    "MATRICOLA ATTUALE".MAGNETE_LAT_DX_ESCLUSO;
      )     ;
      =     "77YV4B";
NETWORK
TITLE =APERTURA BRACCIO MAGNETE LATERALE SX

      U(    ;
      U     "AP&T in Manuale";
      U(    ;
      O     "M137.3";
      O     "M131.0";
      )     ;
      O     ;
      U(    ;
      O     "AP&T in Automatico";
      O     "AP&T in Manuale";
      )     ;
      U(    ;
      O     "C.pacco :ind. magneti";
      O     "C.produz. :ind. magneti";
      )     ;
      )     ;
      UN    "77YV5B";
      =     "77YV5A";
NETWORK
TITLE =CHIUSURA BRACCIO MAGNETE LATERALE SX

      U(    ;
      U     "AP&T in Manuale";
      U     "M137.2";
      O     ;
      U(    ;
      U(    ;
      O     "AP&T in Automatico";
      O     "Singolo";
      )     ;
      U     "AP&T in ciclo";
      O     "AP&T in Manuale";
      )     ;
      U     "M35.6";
      U     "46SQ10";
      )     ;
      UN    "Pacco magnete lat.sx";
      UN    "77YV5A";
      =     "77YV5B";
NETWORK
TITLE =APERTURA BRACCIO MAGNETE LATERALE DX

      U(    ;
      U     "AP&T in Manuale";
      U(    ;
      O     "M137.1";
      O     "M131.0";
      )     ;
      O     ;
      U(    ;
      O     "AP&T in Automatico";
      O     "AP&T in Manuale";
      )     ;
      U(    ;
      O     "C.pacco :ind. magneti";
      O     "C.produz. :ind. magneti";
      )     ;
      )     ;
      UN    "77YV6B";
      =     "77YV6A";
NETWORK
TITLE =CHIUSURA BRACCIO MAGNETE LATERALE DX
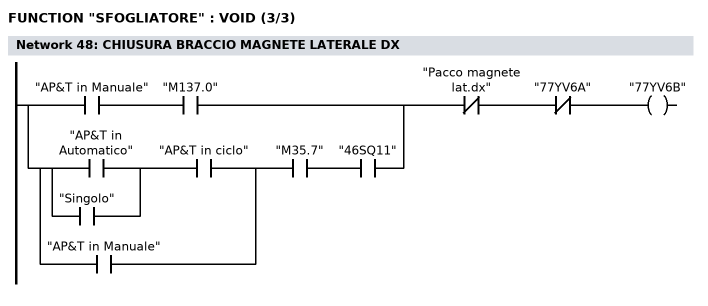
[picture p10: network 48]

      U(    ;
      U     "AP&T in Manuale";
      U     "M137.0";
      O     ;
      U(    ;
      U(    ;
      O     "AP&T in Automatico";
      O     "Singolo";
      )     ;
      U     "AP&T in ciclo";
      O     "AP&T in Manuale";
      )     ;
      U     "M35.7";
      U     "46SQ11";
      )     ;
      UN    "Pacco magnete lat.dx";
      UN    "77YV6A";
      =     "77YV6B";
NETWORK
TITLE =

END_FUNCTION

